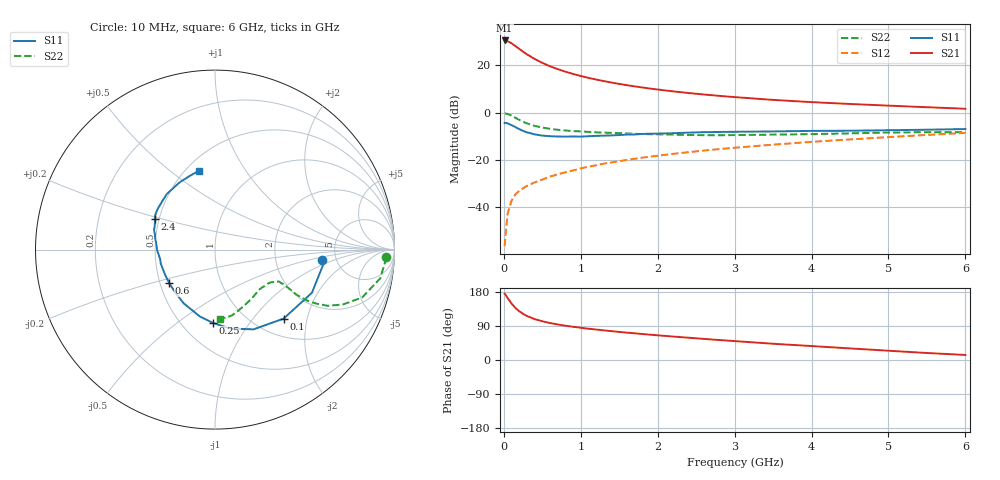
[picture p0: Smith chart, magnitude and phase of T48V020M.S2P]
! Infineon Technologies  Discrete & RF Semiconductors
! BFR182T
! Si NPN RF Bipolar Junction Transistor in SC75
! VCE = 8 V  IC = 20 mA
! Common Emitter S-Parameters:  October  1999
# GHz  S  MA  R  50
!  f  S11  S21  S12  S22
! GHz  MAG  ANG  MAG  ANG  MAG  ANG  MAG  ANG
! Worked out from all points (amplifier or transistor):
!   36 points, 10 MHz to 6 GHz, reference 50 ohm
!   highest |S21| = 30.5 dB at 10 MHz (marker M1)
!   |S21| within 3 dB of that: start of sweep to 176.8 MHz
!   unconditionally stable (mu >= 1): 771.1 MHz to 3.828 GHz
!   at 250 MHz: K = 0.60, MSG = 28.9 dB, |S12| = -32.0 dB
!   at 1.4 GHz: K = 1.08, MAG = 15.2 dB, |S12| = -21.1 dB
!   at 6 GHz: K = 0.87, MSG = 5.1 dB, |S12| = -8.6 dB
!   S11 on the Smith chart (normalised r, x): 10 MHz: 3.85, -0.70; 100 MHz: 1.33, -1.45; 250 MHz: 0.70, -0.69; 600 MHz: 0.56, -0.23; 2.4 GHz: 0.47, +0.19; 6 GHz: 0.58, +0.64
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0.01  0.5986 -5.6  33.41 174.8  0.0015 78.4  0.9544 -2.6
0.02  0.608 -8.2  33.27 172.9  0.0024 91.3  0.952 -3.8
0.05  0.5912 -24.0  32.17 163.2  0.0074 84.9  0.9343 -9.9
0.1  0.5421 -45.2  29.06 149.1  0.0137 75.2  0.8624 -18.0
0.15  0.4935 -64.2  25.48 137.4  0.0187 67.7  0.7744 -23.3
0.2  0.4477 -79.2  22.18 128.6  0.0222 66.8  0.7014 -26.5
0.25  0.409 -91.4  19.34 121.7  0.0251 63.4  0.6382 -28.1
0.3  0.3826 -102.6  17.02 116.2  0.0282 63.2  0.5916 -28.9
0.4  0.3463 -120.4  13.59 107.9  0.0334 63.6  0.5222 -29.0
0.5  0.3256 -132.9  11.23 102.2  0.0384 64.9  0.4824 -28.1
0.6  0.3162 -143.6  9.519 97.5  0.0443 66.1  0.4536 -27.5
0.8  0.3101 -159.3  7.317 90.5  0.0544 67.9  0.4179 -26.8
0.9  0.3121 -165.3  6.539 87.7  0.0597 68.9  0.4053 -26.7
1.1  0.3159 -175.5  5.413 82.5  0.0717 69.3  0.3901 -27.1
1.3  0.3254 177.2  4.623 78.2  0.0834 69.8  0.3767 -28.2
1.6  0.342 168.0  3.785 72.2  0.0997 69.7  0.3613 -30.3
2.2  0.366 156.2  2.807 61.9  0.134 68.8  0.3418 -36.7
2.4  0.3764 152.9  2.589 58.8  0.1455 68.3  0.3356 -39.1
3.5  0.3991 137.2  1.852 42.9  0.2097 63.9  0.3418 -53.9
4.5  0.413 125.2  1.519 30.6  0.2705 58.7  0.363 -68.6
5.5  0.4337 109.1  1.297 18.5  0.3368 53.0  0.3841 -80.9
6  0.4487 101.4  1.204 13.3  0.3712 49.4  0.385 -85.7
